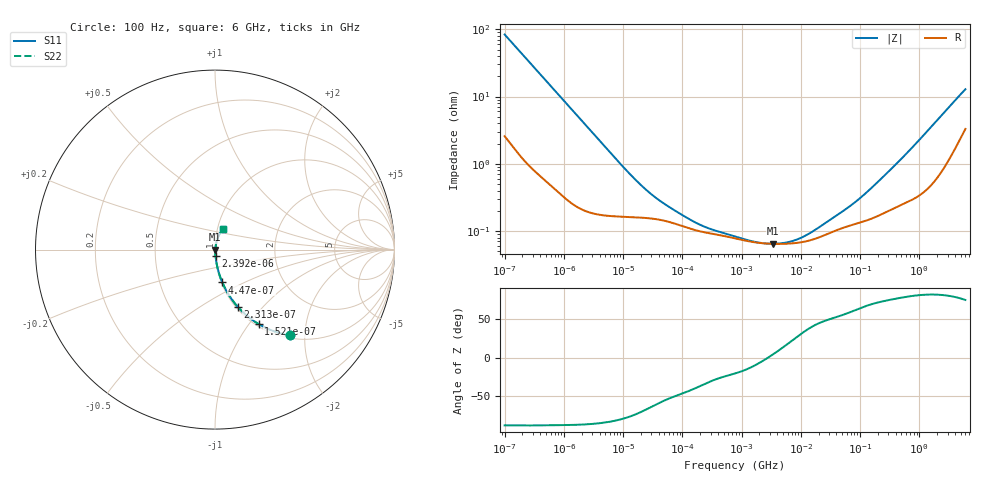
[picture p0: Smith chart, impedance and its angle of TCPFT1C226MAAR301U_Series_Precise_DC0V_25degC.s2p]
! TCPFT1C226MAAR301U Polymer Tantalum Capacitor Sparameter Model
! Model Generated by Samsung Electro-Mechanics
! Samsung Sparameter Version 5.0
! Date : Oct-21-2025
! Products : Polymer Tantalum Capacitor
! Characteristics :
!  Nominal Capacitance = 22uF
!  Capacitance Tolerance = +/-20%
!  ESR = 300 mohm max at 100kHz
!  Rated Voltage = 16Vdc
!  Size = 1206(unit:inch), 3216(unit:mm)
!  Length = 3.20+/-0.20mm
!  Width = 1.60+/-0.20mm
!  Thickness = 0.70+/-0.10mm
!  Lineup = Conductive Polymer Type
!  Feature = PFT
!  Measurement Temperature : 25degC.
!  DC bias Value = 0V
!  Frequency : 100Hz ~ 6GHz
! External Node Assignments :
!  1  o---||---o  2
# MHz S RI R 50.0
! Freq.  Real(S11)  Im(S11)  Real(S12)  Im(S12)  Real(S21)  Im(S21)  Real(S22)  Im(S22)
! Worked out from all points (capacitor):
!   300 points, 100 Hz to 6 GHz, reference 50 ohm
!   read as one part in series: C = 18.9 uF near 106.2 Hz
!   lowest |Z| = 64.6 mohm at 3.361 MHz (marker M1)
!   series resonance near 2.8 MHz, so ESL is about 170 pH
!   S11 on the Smith chart (normalised r, x): 100 Hz: 1.05, -1.68; 152.1 Hz: 1.03, -1.11; 231.3 Hz: 1.02, -0.74; 447 Hz: 1.01, -0.38; 2.392 kHz: 1.00, -0.07; 6 GHz: 1.07, +0.25
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0.0001  0.4155 -0.4777  0.5845 0.4777  0.5845 0.4777  0.4155 -0.4777
0.0001520888  0.2424 -0.4144  0.7576 0.4144  0.7576 0.4144  0.2424 -0.4144
0.00023131  0.1259 -0.318  0.8741 0.318  0.8741 0.318  0.1259 -0.318
0.0004470407  0.0409 -0.1831  0.9591 0.1831  0.9591 0.1831  0.0409 -0.1831
0.0008639723  0.0134 -0.0988  0.9866 0.0988  0.9866 0.0988  0.0134 -0.0988
0.001998454  0.004 -0.0436  0.996 0.0436  0.996 0.0436  0.004 -0.0436
0.00239186  0.00329 -0.0365  0.9967 0.0365  0.9967 0.0365  0.00329 -0.0365
0.01442621  0.00164 -0.0062  0.9984 0.0062  0.9984 0.0062  0.00164 -0.0062
0.02473303  0.00157 -0.00375  0.9984 0.00375  0.9984 0.00375  0.00157 -0.00375
0.03993819  0.00148 -0.00249  0.9985 0.00249  0.9985 0.00249  0.00148 -0.00249
0.09238102  0.00121 -0.00133  0.9988 0.00133  0.9988 0.00133  0.00121 -0.00133
0.1895612  0.000999 -0.000773  0.999 0.000773  0.999 0.000773  0.000999 -0.000773
0.3249932  0.000906 -0.000519  0.9991 0.000519  0.9991 0.000519  0.000906 -0.000519
0.7981464  0.000773 -0.000286  0.9992 0.000286  0.9992 0.000286  0.000773 -0.000286
1.738854  0.000675 -0.000112  0.9993 0.000112  0.9993 0.000112  0.000675 -0.000112
3.360592  0.000644 4.51e-05  0.9994 -4.51e-05  0.9994 -4.51e-05  0.000644 4.51e-05
7.321436  0.000656 0.000277  0.9993 -0.000277  0.9993 -0.000277  0.000656 0.000277
15.95059  0.000747 0.000646  0.9993 -0.000646  0.9993 -0.000646  0.000747 0.000646
80.38067  0.00126 0.00231  0.9987 -0.00231  0.9987 -0.00231  0.00126 0.00231
318.7652  0.00209 0.00772  0.9979 -0.00772  0.9979 -0.00772  0.00209 0.00772
1705.531  0.00653 0.0372  0.9935 -0.0372  0.9935 -0.0372  0.00653 0.0372
6000  0.0458 0.1148  0.9542 -0.1148  0.9542 -0.1148  0.0458 0.1148
